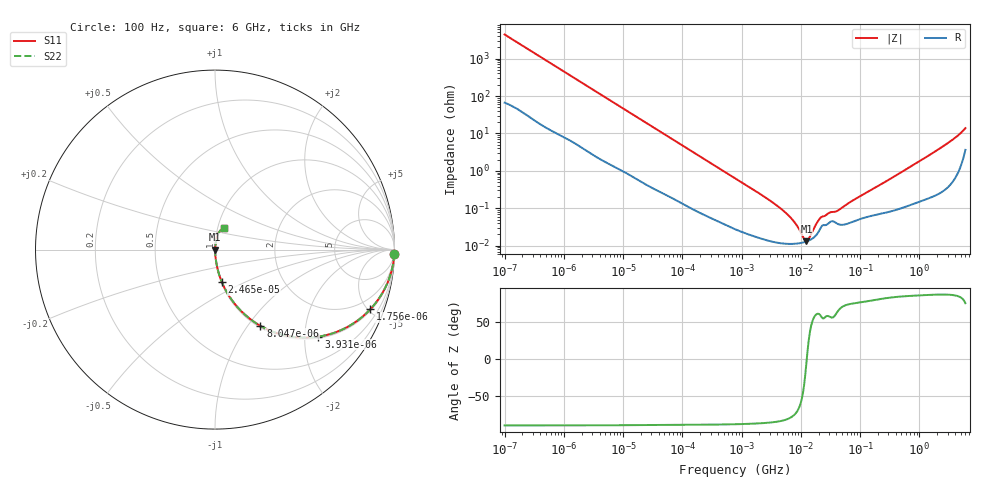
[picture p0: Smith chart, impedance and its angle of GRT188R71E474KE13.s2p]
!Murata Part Number: GRT188R71E474KE13
!These Parameters are Measured in Series Mode Connection
!Data Generated on Jun 19, 2026
!  o--ll--o
!Port1  Port2
!  o------o
!Operation Temp=25[degC], DC Bias Voltage=0[V]
!Freq. Start=100[Hz] Stop=6[GHz] 401[Steps]
# Hz S RI R 50
!Freq.(Hz) S11(Real) S11(Imag) S21(Real) S21(Imag) S12(Real) S12(Imag) S22(Real) S22(Imag)
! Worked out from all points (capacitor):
!   401 points, 100 Hz to 6 GHz, reference 50 ohm
!   read as one part in series: C = 360 nF near 109 Hz
!   lowest |Z| = 13 mohm at 12.44 MHz (marker M1)
!   series resonance near 12.61 MHz, so ESL is about 440 pH
!   S11 on the Smith chart (normalised r, x): 100 Hz: 2, -88; 1.756 kHz: 1.10, -5.18; 3.931 kHz: 1.04, -2.34; 8.047 kHz: 1.02, -1.15; 24.65 kHz: 1.01, -0.38; 6 GHz: 1.07, +0.27
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100  0.9991 -0.0227  0.000856 0.0227  0.000856 0.0227  0.9991 -0.0227
501  0.986 -0.1099  0.014 0.1099  0.014 0.1099  0.986 -0.1099
1756  0.8659 -0.3317  0.1341 0.3317  0.1341 0.3317  0.8659 -0.3317
2008  0.833 -0.364  0.167 0.364  0.167 0.364  0.833 -0.364
3931  0.5757 -0.4852  0.4243 0.4852  0.4243 0.4852  0.5757 -0.4852
8047  0.2529 -0.4247  0.7471 0.4247  0.7471 0.4247  0.2529 -0.4247
13169  0.1165 -0.3103  0.8835 0.3103  0.8835 0.3103  0.1165 -0.3103
24648  0.0389 -0.1825  0.9611 0.1825  0.9611 0.1825  0.0389 -0.1825
40335  0.0163 -0.115  0.9837 0.115  0.9837 0.115  0.0163 -0.115
774597  0.000317 -0.00641  0.9997 0.00641  0.9997 0.00641  0.000317 -0.00641
5311619  0.000114 -0.000801  0.9999 0.000801  0.9999 0.000801  0.000114 -0.000801
7599586  0.000112 -0.000436  0.9999 0.000436  0.9999 0.000436  0.000112 -0.000436
1.137099e7  0.000124 -8.65e-05  0.9999 8.65e-05  0.9999 8.65e-05  0.000124 -8.65e-05
1.243624e7  0.00013 -1.15e-05  0.9999 1.15e-05  0.9999 1.15e-05  0.00013 -1.15e-05
1.360128e7  0.000137 6.43e-05  0.9999 -6.43e-05  0.9999 -6.43e-05  0.000137 6.43e-05
1.555665e7  0.000154 0.000181  0.9998 -0.000181  0.9998 -0.000181  0.000154 0.000181
1.946e7  0.000221 0.000393  0.9998 -0.000393  0.9998 -0.000393  0.000221 0.000393
2.225763e7  0.000323 0.000488  0.9997 -0.000488  0.9997 -0.000488  0.000323 0.000488
4.165952e7  0.000385 0.000768  0.9996 -0.000768  0.9996 -0.000768  0.000385 0.000768
3.124326e8  0.000841 0.00585  0.9992 -0.00585  0.9992 -0.00585  0.000841 0.00585
2.34314e9  0.00438 0.0416  0.9956 -0.0416  0.9956 -0.0416  0.00438 0.0416
6e9  0.0508 0.1223  0.9492 -0.1223  0.9492 -0.1223  0.0508 0.1223
